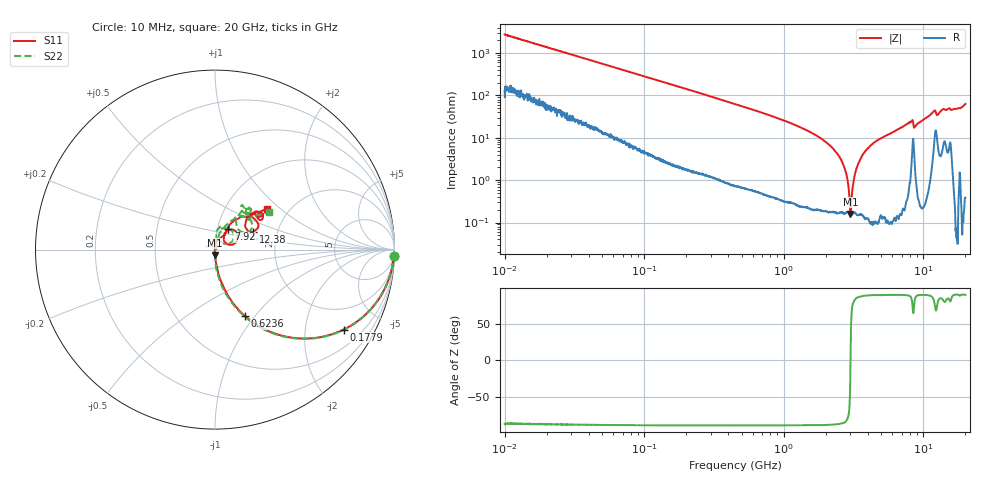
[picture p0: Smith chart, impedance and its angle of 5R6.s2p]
!Keysight Technologies,P5008B,MY61100088,A.16.20.02
!Date: Friday, August 30, 2024 13:08:03
!Correction: S11(C  2-Port  )
!S21(C  2-Port  )
!S12(C  2-Port  )
!S22(C  2-Port  )
!S2P File: Measurements: S11, S21, S12, S22:Log Frequency Sweep
# Hz S  dB  R 50
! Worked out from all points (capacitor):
!   1601 points, 10 MHz to 20 GHz, reference 50 ohm
!   read as one part in series: C = 5.8 pF near 10.39 MHz
!   lowest |Z| = 160 mohm at 3.005 GHz (marker M1)
!   series resonance near 3.006 GHz, so ESL is about 480 pH
!   S11 on the Smith chart (normalised r, x): 10 MHz: 3, -55; 177.9 MHz: 1.03, -3.19; 623.6 MHz: 1.00, -0.89; 7.92 GHz: 1.13, +0.26; 12.38 GHz: 1.50, +0.32; 20 GHz: 1.56, +0.81
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1e7  -0.02 -2.1  -28.80 85.2  -28.80 85.2  -0.02 -2.1
3.555162e7  -0.10 -7.3  -18.00 81.0  -18.00 81.0  -0.10 -7.3
1.263918e8  -0.83 -24.0  -7.86 65.2  -7.87 65.2  -0.83 -24.0
1.779365e8  -1.48 -31.9  -5.57 57.3  -5.58 57.3  -1.48 -32.0
4.472136e8  -5.49 -57.5  -1.50 31.6  -1.51 31.6  -5.49 -57.9
6.236416e8  -7.82 -65.7  -0.83 23.3  -0.83 23.3  -7.83 -66.3
1.589917e9  -16.99 -81.6  -0.10 6.6  -0.11 6.6  -16.98 -83.5
2.473129e9  -24.22 -87.3  -0.03 0.8  -0.03 0.8  -24.10 -87.5
3.004939e9  -30.64 -91.3  -0.01 -1.7  -0.02 -1.8  -30.20 -84.7
3.33599e9  -37.32 -97.1  -0.01 -3.1  -0.01 -3.1  -36.04 -75.4
3.514952e9  -44.33 -94.8  -0.01 -3.8  -0.01 -3.8  -41.34 -62.9
3.616581e9  -63.50 120.7  -0.01 -4.1  -0.01 -4.2  -46.47 -18.6
3.721149e9  -43.18 116.7  -0.01 -4.6  -0.01 -4.6  -41.60 23.9
3.865292e9  -39.69 106.9  -0.00 -5.1  -0.01 -5.2  -38.80 44.8
4.25055e9  -32.28 89.6  -0.00 -6.4  -0.01 -6.5  -32.19 69.6
5.652411e9  -25.90 76.0  -0.00 -10.9  -0.01 -11.0  -25.49 77.2
7.91985e9  -17.31 56.8  -0.10 -18.8  -0.11 -19.0  -17.63 77.1
8.834242e9  -22.39 51.1  -0.08 -18.4  -0.08 -18.5  -22.91 72.4
1.163675e10  -12.42 50.0  -0.42 -31.0  -0.43 -31.2  -12.67 53.3
1.237806e10  -12.63 25.3  -1.18 -27.2  -1.18 -27.4  -14.40 30.3
1.661757e10  -10.55 42.3  -0.37 -38.4  -0.37 -38.7  -10.76 58.3
2e10  -8.69 37.6  -0.62 -53.0  -0.62 -53.3  -8.68 34.9
